(* Logix 5000 Routine export DH485Router; software revision 19.01 *)

TYPE AparianDH485ROutput :
STRUCT
   RoutingInhibit : BOOL;
END_STRUCT
END_TYPE

TYPE AparianDH485RMsgDataType :
STRUCT
   BOOLEAN : BOOL;
   INT : BOOL;
   REAL : BOOL;
END_STRUCT
END_TYPE

TYPE AparianDH485RInput :
STRUCT
   Instance : STRING;
   Status : AparianDH485RDH485Status;
   TransactionRate : DINT;
   Temperature : REAL;
   DH485RxPacketCount : DINT;
   DH485TxPacketCount : DINT;
   DH485ChecksumErrors : DINT;
   PCCCRequests : DINT;
   PCCCFailures : DINT;
   TagReads : DINT;
   TagWrites : DINT;
   TagConnectionFailures : DINT;
   TagErrors : DINT;
END_STRUCT
END_TYPE

TYPE AparianDH485RDH485Status :
STRUCT
   TransparentPCCCMode : BOOL;
   ReactiveTagMode : BOOL;
   ScheduledTagMode : BOOL;
   UnscheduledMode : BOOL;
   ConfigurationValid : BOOL;
   RoutingInhibited : BOOL;
   Reserved1 : BOOL;
   Reserved2 : BOOL;
   ScheduledTagStatus0 : BOOL;
   ScheduledTagStatus1 : BOOL;
   ScheduledTagStatus2 : BOOL;
   ScheduledTagStatus3 : BOOL;
   ScheduledTagStatus4 : BOOL;
   ScheduledTagStatus5 : BOOL;
   ScheduledTagStatus6 : BOOL;
   ScheduledTagStatus7 : BOOL;
   ScheduledTagStatus8 : BOOL;
   ScheduledTagStatus9 : BOOL;
   ScheduledTagStatus10 : BOOL;
   ScheduledTagStatus11 : BOOL;
   ScheduledTagStatus12 : BOOL;
   ScheduledTagStatus13 : BOOL;
   ScheduledTagStatus14 : BOOL;
   ScheduledTagStatus15 : BOOL;
   ScheduledTagStatus16 : BOOL;
   ScheduledTagStatus17 : BOOL;
   ScheduledTagStatus18 : BOOL;
   ScheduledTagStatus19 : BOOL;
END_STRUCT
END_TYPE

TYPE AparianDH485RMsgResponse :
STRUCT
   Status : INT;
   ResponseLength : INT;
   ResponseData : INT[128];
END_STRUCT
END_TYPE

TYPE AparianDH485RMsgRequest :
STRUCT
   DestinationNode : SINT;
   DF1DataFileAddress : STRING;
   Function : AparianDH485RMsgFunctionType;
   DataType : AparianDH485RMsgDataType;
   ElementCount : INT;
   RequestData : INT[128];
END_STRUCT
END_TYPE

TYPE AparianDH485RMsgFunctionType :
STRUCT
   PLC5TypedRead : BOOL;
   PLC5TypedWrite : BOOL;
   SLCTypedRead : BOOL;
   SLCTypedWrite : BOOL;
END_STRUCT
END_TYPE

VAR_GLOBAL   (* controller tags *)
   DH485RMsgeResponse : AparianDH485RMsgResponse;
   DH485R01Input : AparianDH485RInput := (Instance := 'South', Status.ReactiveTagMode := 1, Status.ConfigurationValid := 1, TransactionRate := 31, Temperature := 46.3, DH485RxPacketCount := 34218, DH485TxPacketCount := 34217, TagReads := 16522, TagWrites := 587);
   DH485RMsgRequest : AparianDH485RMsgRequest := (DestinationNode := 5, DF1DataFileAddress := 'N10:0', Function.PLC5TypedRead := 1, DataType.INT := 1, ElementCount := 16);
   DH485RMsgTrigger : BOOL;
   DH485RMessage : MESSAGE;
        MessageParameters(MessageType := CIP Generic, RequestedLength := 360, ConnectedFlag := 2, ConnectionPath := DH485R01, ServiceCode := 16#006a, ObjectType := 16#0408, TargetObject := 1, LocalElement := DH485RMsgRequest, DestinationTag := DH485RMsgeResponse)
   DH485R01Output : AparianDH485ROutput;
END_VAR

PROGRAM MainProgram

ROUTINE DH485Router   (* ladder *)
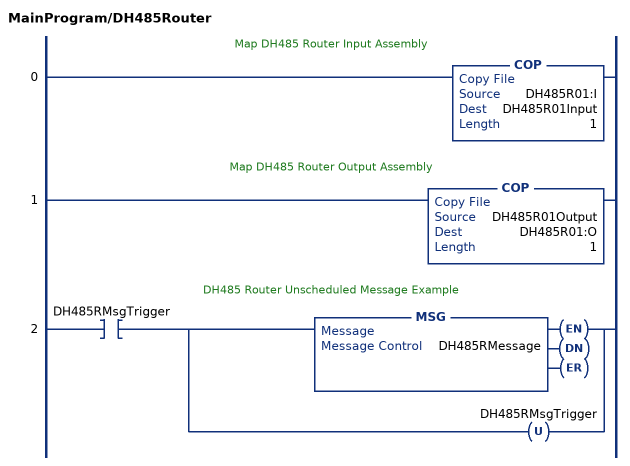
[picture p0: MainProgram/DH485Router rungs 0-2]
   // Map DH485 Router Input Assembly
   0: COP(DH485R01:I,DH485R01Input,1);
   // Map DH485 Router Output Assembly
   1: COP(DH485R01Output,DH485R01:O,1);
   // DH485 Router Unscheduled Message Example
   2: XIC(DH485RMsgTrigger)[MSG(DH485RMessage) ,OTU(DH485RMsgTrigger) ];
END_ROUTINE
END_PROGRAM
